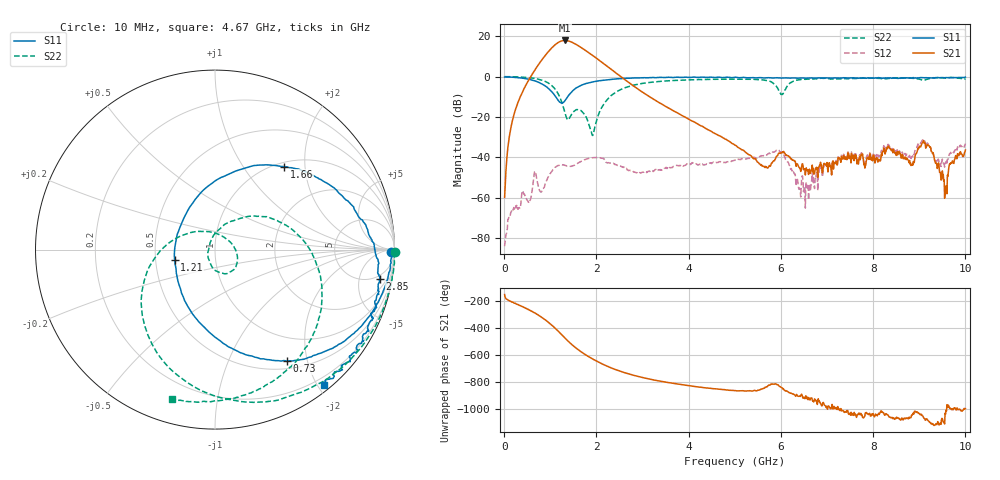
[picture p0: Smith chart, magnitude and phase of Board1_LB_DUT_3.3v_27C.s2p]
! Created Tue May 27 15:28:40 2025
# hz S ma R 50
! 2 Port Network Data from SP1.SP block
! freq  magS11  angS11  magS21  angS21  magS12  angS12  magS22  angS22
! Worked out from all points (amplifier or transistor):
!   1000 points, 10 MHz to 10 GHz, reference 50 ohm
!   highest |S21| = 17.9 dB at 1.31 GHz (marker M1)
!   |S21| within 3 dB of that: 1.063 GHz to 1.635 GHz (572.3 MHz wide, 42.4 % of centre)
!   unconditionally stable (mu >= 1): 58.67 MHz to 61.88 MHz; 90.49 MHz to 107.9 MHz; 111.9 MHz to end of sweep
!   at 1.67 GHz: K = 7.39, MAG = 16.5 dB, |S12| = -41.9 dB
!   at 5.01 GHz: K = 43.81, MAG = -15.7 dB, |S12| = -41.4 dB
!   at 10 GHz: K = 15.32, MAG = -16.5 dB, |S12| = -33.1 dB
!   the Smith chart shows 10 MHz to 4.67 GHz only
!   S11 on the Smith chart (normalised r, x): 10 MHz: 63, -46; 730 MHz: 0.61, -1.67; 1.21 GHz: 0.63, -0.08; 1.66 GHz: 1.08, +1.57; 2.85 GHz: 4, -10; 4.67 GHz: 0.09, -2.09
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1e7  0.9796 -0.9  0.001022 -154.8  6.331e-05 137.8  1.005 -0.8
2.1e8  0.9646 -14.4  0.1115 144.0  0.0005744 76.8  0.9953 -18.7
7.3e8  0.7396 -57.1  1.897 55.4  0.002172 55.2  0.8774 -75.9
9e8  0.5777 -77.7  3.45 15.5  0.002376 112.8  0.7537 -102.2
1.04e9  0.4134 -102.5  5.267 -23.4  0.004662 101.3  0.5902 -130.4
1.13e9  0.3055 -127.6  6.516 -52.1  0.005958 87.0  0.4488 -153.3
1.21e9  0.2322 -165.6  7.41 -79.4  0.006527 74.2  0.3051 -178.8
1.31e9  0.2464 134.9  7.889 -114.4  0.006414 61.1  0.139 133.0
1.46e9  0.4134 82.4  7.202 -163.5  0.00602 57.7  0.1155 -1.0
1.66e9  0.6027 50.1  5.345 142.7  0.007839 53.4  0.1456 -67.4
1.68e9  0.6163 47.8  5.162 138.0  0.008099 51.7  0.1393 -71.4
1.88e9  0.7266 30.5  3.602 95.0  0.009561 33.0  0.04731 -149.1
2.08e9  0.7985 18.4  2.456 58.3  0.009736 11.2  0.146 70.0
2.41e9  0.877 3.4  1.268 9.5  0.006713 -7.0  0.4026 21.2
2.85e9  0.9317 -10.1  0.5435 -37.3  0.00424 -5.3  0.6332 -19.9
3.34e9  0.9516 -23.4  0.2342 -74.3  0.004864 10.6  0.7579 -51.0
4.67e9  0.9669 -51.1  0.03435 -136.7  0.007848 -4.5  0.8638 -106.1
5.01e9  0.9683 -57.8  0.02013 -146.8  0.008528 -9.0  0.8685 -117.9
6.67e9  0.9318 -90.0  0.005204 158.8  0.002873 161.8  0.8735 -148.5
8.34e9  0.9254 -136.3  0.0187 20.4  0.02033 29.3  0.9016 172.4
9.57e9  0.9488 -169.0  0.001272 38.0  0.007014 55.2  0.9239 162.4
1e10  0.975 177.4  0.01522 79.2  0.02202 70.2  0.8965 155.9
